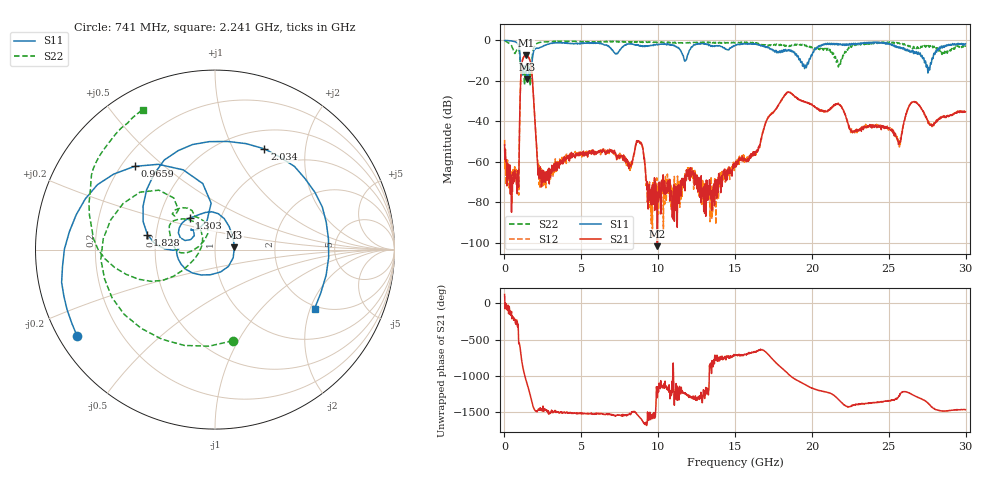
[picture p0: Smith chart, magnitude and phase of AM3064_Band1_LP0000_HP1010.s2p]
# Hz S DB R 50.0
!freq dBS11 angS11 dBS21 angS21 dBS12 angS12 dBS22 angS22
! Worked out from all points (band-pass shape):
!   1600 points, 10 MHz to 29.98 GHz, reference 50 ohm
!   highest |S21| = -7.45 dB at 1.397 GHz (marker M1); lowest = -101.7 dB at 9.944 GHz (marker M2)
!   |S21| within 3 dB of the highest: 1.156 GHz to 1.68 GHz (523.9 MHz wide, 37 % of centre)
!   lowest |S11| = -19.3 dB at 1.472 GHz (marker M3), VSWR 1.24, Z = 62.1 + j1.49 ohm
!   |S11| at or under -10 dB: 1.031 GHz to 1.804 GHz (772.9 MHz wide, 54.5 % of centre); 19.25 GHz to 19.81 GHz (557.3 MHz wide, 2.85 % of centre); 27.3 GHz to 27.79 GHz (490.5 MHz wide, 1.78 % of centre)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
!   |S22| runs from -22.4 to -0.3 dB; largest |S21 - S12| = 0.0049
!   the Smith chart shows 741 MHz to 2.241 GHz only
!   S11 on the Smith chart (normalised r, x): 741 MHz: 0.05, -0.29; 965.9 MHz: 0.25, +0.40; 1.303 GHz: 0.71, +0.26; 1.828 GHz: 0.45, +0.09; 2.034 GHz: 0.72, +1.34; 2.241 GHz: 1.91, -2.15
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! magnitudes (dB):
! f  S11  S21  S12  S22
! 10 MHz  -0.1  -51.7  -49.2  -0.3
! 741 MHz  -0.8  -68.1  -69.1  -5.7
! 965.9 MHz  -3.8  -49.6  -49.8  -5.6
! 1.135 GHz  -16.1  -11.4  -11.4  -12.0
! 1.303 GHz  -12.9  -7.7  -7.6  -22.2
! 1.397 GHz  -13.9  -7.4  -7.5  -13.2
! 1.472 GHz  -19.3  -7.6  -7.6  -11.1
! 1.828 GHz  -8.3  -20.5  -20.5  -6.8
! 2.034 GHz  -4.1  -46.5  -46.6  -1.9
! 2.241 GHz  -3.8  -64.3  -71.3  -1.1
! 5.015 GHz  -1.4  -55.8  -55.9  -0.8
! 8.763 GHz  -2.8  -50.2  -50.1  -1.1
! 9.401 GHz  -2.6  -76.4  -75.8  -0.9
! 9.944 GHz  -2.2  -101.7  -75.7  -1.0
! 10 GHz  -2.0  -75.7  -74.8  -0.9
! 13.64 GHz  -2.9  -76.7  -77.6  -1.2
! 15 GHz  -2.5  -61.3  -61.4  -1.2
! 18.34 GHz  -5.4  -26.0  -26.0  -2.8
! 19.99 GHz  -7.6  -31.9  -31.9  -3.4
! 25 GHz  -1.5  -43.5  -43.7  -1.1
! 27.56 GHz  -15.9  -40.4  -41.0  -2.8
! 29.98 GHz  -1.7  -35.3  -35.6  -3.2
